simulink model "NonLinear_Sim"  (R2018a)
settings: Solver=ode113  StartTime=0.0  StopTime=40  FixedStep=Ts  MaxStep=0.005  RelTol=1e-5  EnableMultiTasking=on
InitFcn:
  | init
StopFcn:
  | pl
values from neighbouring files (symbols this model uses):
  d2r = pi/180    (= 0.0174532925199)    [init.m]    (also in LQR_Design.m)
  Ixx = 2330    [init.m]
  Iyy = 18829    [init.m]
  Izz = 18670    [init.m]
  Thr = 3.0    (= 3)    [init.m]
  x1_ini = [-1,0, -2,0, 2,0]*d2r    [init.m]
  x2_ini = [x1_ini,x2_ini]    [init.m]
  Xcg = 92.1    [init.m]
undefined symbols (not defined in the file or in its folder): Av, Bv, Cv, Dv, Kmix, Kq

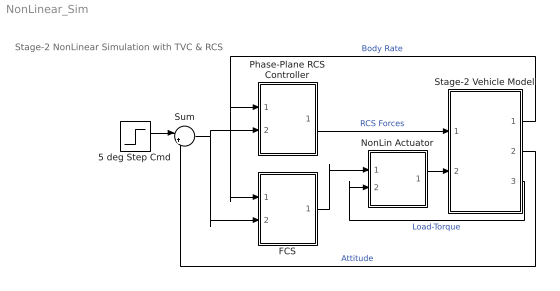
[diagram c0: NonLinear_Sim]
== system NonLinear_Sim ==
  note: Stage-2 NonLinear Simulation with TVC & RCS
  5 deg Step Cmd : Step  Time=0  Before=[0,0,0]  After=[1, 1, -1]*d2r*5  SampleTime=0
  FCS : Subsystem
  NonLin Actuator : Subsystem
  Phase-Plane RCS Controller : Subsystem
  Stage-2 Vehicle Model : Subsystem
  Sum : Sum  Inputs=|+-
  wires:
  Stage-2 Vehicle Model/1(Wb) -> FCS/1(rate), Phase-Plane RCS Controller/1(rate)  "Body Rate"
  Sum/1 -> FCS/2(atter), Phase-Plane RCS Controller/2(atter)
  Phase-Plane RCS Controller/1(f(i)) -> Stage-2 Vehicle Model/1(Frcs)  "RCS Forces"
  Stage-2 Vehicle Model/2(atti) -> Sum/2  "Attitude"
  NonLin Actuator/1(del) -> Stage-2 Vehicle Model/2(dy,dz)
  Stage-2 Vehicle Model/3(TL) -> NonLin Actuator/2(TL)  "Load-Torque"
  FCS/1(DQ,DR) -> NonLin Actuator/1(dc)
  5 deg Step Cmd/1 -> Sum/1

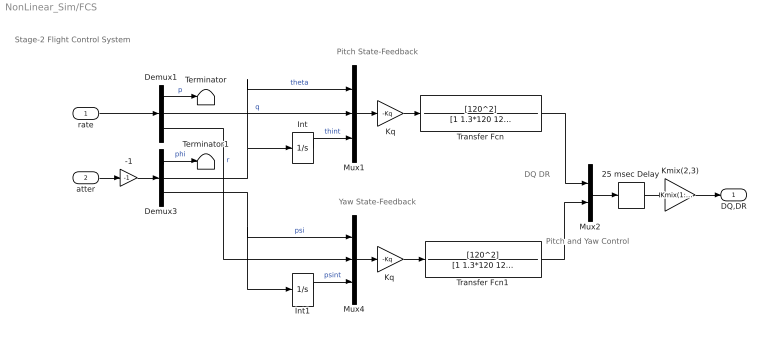
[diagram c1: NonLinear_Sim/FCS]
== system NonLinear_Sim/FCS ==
  note: Stage-2 Flight Control System
  note: DQ DR
  note: Pitch State-Feedback
  note: Yaw State-Feedback
  note: Pitch and Yaw Control
  rate : Inport
  atter : Inport  Port=2
  -1 : Gain  Gain=-1
  25 msec Delay : TransportDelay  DelayTime="[1  1]*0.025"  InitialOutput=[0 0]  PadeOrder=2
  Demux1 : Demux  Outputs=3
  Demux3 : Demux  Outputs=3
  Int : Integrator
  Int1 : Integrator
  Kmix(2,3) : Gain  Gain=Kmix(1:2,2:3)  Multiplication=Matrix(K*u)
  Kq : Gain  Gain=-Kq  Multiplication=Matrix(K*u)
  "Kq " : Gain  Gain=-Kq  Multiplication=Matrix(K*u)
  Mux1 : Mux  Inputs=3
  Mux2 : Mux  Inputs=2
  Mux4 : Mux  Inputs=3
  Terminator : Terminator
  Terminator1 : Terminator
  Transfer Fcn : TransferFcn  Numerator=[120^2]  Denominator=[1 1.3*120 120^2]
  Transfer Fcn1 : TransferFcn  Numerator=[120^2]  Denominator=[1 1.3*120 120^2]
  DQ,DR : Outport
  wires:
  25 msec Delay/1 -> Kmix(2,3)/1
  Transfer Fcn1/1 -> Mux2/2
  Kq/1 -> Transfer Fcn/1
  Mux2/1 -> 25 msec Delay/1
  "Kq "/1 -> Transfer Fcn1/1
  Transfer Fcn/1 -> Mux2/1
  Demux3/1 -> Terminator1/1  "phi"
  Demux1/1 -> Terminator/1  "p"
  Kmix(2,3)/1 -> DQ,DR/1
  rate/1 -> Demux1/1
  Demux3/2 -> Mux1/1, Int/1  "theta"
  Demux1/2 -> Mux1/2  "q"
  Int/1 -> Mux1/3  "thint"
  Int1/1 -> Mux4/3  "psint"
  Demux1/3 -> Mux4/2  "r"
  Demux3/3 -> Mux4/1, Int1/1  "psi"
  Mux1/1 -> Kq/1
  Mux4/1 -> "Kq "/1
  atter/1 -> -1/1
  -1/1 -> Demux3/1

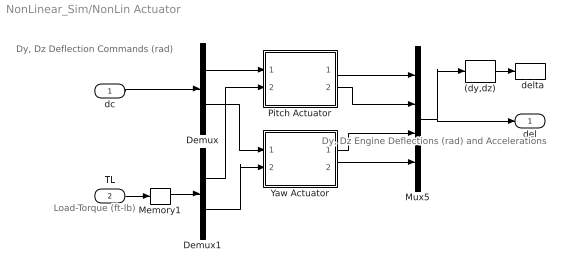
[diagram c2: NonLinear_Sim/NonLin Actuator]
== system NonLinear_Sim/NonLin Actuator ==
  note: Dy, Dz Engine Deflections (rad) and Accelerations
  note: Dy, Dz Deflection Commands (rad)
  note: Load-Torque (ft-lb)
  dc : Inport
  TL : Inport  Port=2
  "  delta" : ToWorkspace  VariableName=delta  SampleTime=-1
  (dy,dz) : Selector  InputPortWidth=4  IndexOptions=Index vector (dialog)  Indices=[1,3]  OutputSizes=1
  Demux : Demux  Outputs=2
  Demux1 : Demux  Outputs=2
  Memory1 : Memory
  Mux5 : Mux
  Pitch Actuator : Subsystem
  Yaw Actuator : Subsystem
  del : Outport
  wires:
  Pitch Actuator/1(del) -> Mux5/1
  Yaw Actuator/1(del) -> Mux5/3
  Memory1/1 -> Demux1/1
  (dy,dz)/1 -> "  delta"/1
  Demux1/1 -> Pitch Actuator/2(TL)
  Mux5/1 -> (dy,dz)/1, del/1
  Demux1/2 -> Yaw Actuator/2(TL)
  Demux/2 -> Yaw Actuator/1(delc)
  Pitch Actuator/2(ddot) -> Mux5/2
  Demux/1 -> Pitch Actuator/1(delc)
  Yaw Actuator/2(ddot) -> Mux5/4
  dc/1 -> Demux/1
  TL/1 -> Memory1/1

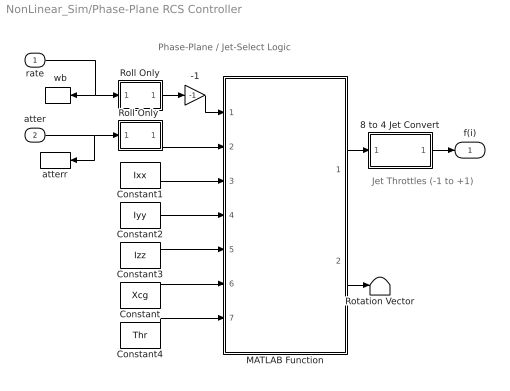
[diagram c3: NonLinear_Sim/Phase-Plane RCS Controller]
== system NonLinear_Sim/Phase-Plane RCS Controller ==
  note: Jet Throttles (-1 to +1)
  note: Phase-Plane / Jet-Select Logic
  rate : Inport
  atter : Inport  Port=2
  "  wb" : ToWorkspace  VariableName=wb  SampleTime=-1
  -1 : Gain  Gain=-1
  8 to 4 Jet Convert : Subsystem
  Constant : Constant  Value=Xcg
  Constant1 : Constant  Value=Ixx
  Constant2 : Constant  Value=Iyy
  Constant3 : Constant  Value=Izz
  Constant4 : Constant  Value=Thr
  MATLAB Function : MATLAB Function  TreatAsAtomicUnit=on
  Roll Only : Subsystem
  "Roll Only " : Subsystem
  Rotation Vector : Terminator
  atterr : ToWorkspace  VariableName=atter  SampleTime=-1
  f(i) : Outport
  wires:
  atter/1 -> atterr/1, "Roll Only "/1(w)
  "Roll Only "/1(p) -> MATLAB Function/2(Atter)
  Roll Only/1(p) -> -1/1
  -1/1 -> MATLAB Function/1(Rater)
  Constant/1 -> MATLAB Function/6(Xcg)
  rate/1 -> Roll Only/1(w), "  wb"/1
  Constant1/1 -> MATLAB Function/3(J11)
  Constant2/1 -> MATLAB Function/4(J22)
  MATLAB Function/1(fp) -> 8 to 4 Jet Convert/1(f(8))
  8 to 4 Jet Convert/1(f(4)) -> f(i)/1
  Constant3/1 -> MATLAB Function/5(J33)
  Constant4/1 -> MATLAB Function/7(Thr)
  MATLAB Function/2(eu) -> Rotation Vector/1

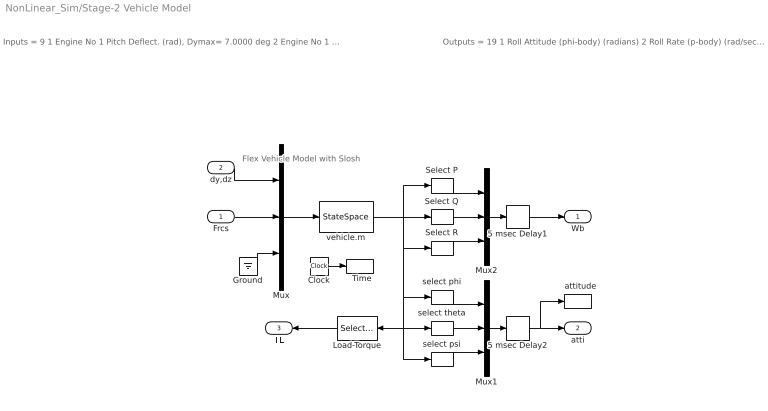
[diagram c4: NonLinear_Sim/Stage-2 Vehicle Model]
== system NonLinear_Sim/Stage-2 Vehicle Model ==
  note: Flex Vehicle Model with Slosh
  note: Outputs = 19 1 Roll Attitude (phi-body) (radians) 2 Roll Rate (p-body) (rad/sec) 3 Pitch Attitude (thet-bdy) (radians) 4 Pitch Rate (q-body) (rad/sec) 5 Yaw Attitude (psi-body) (radians) 6 Yaw Rate (r-body) (rad/sec) 7 Angle of attack, alfa, (radians) 8 Angle of sideslip, beta, (radian) 9 Change in Altitude, delta-h, (feet) 10 Forward Acceleration (V-dot) (ft/sec) 11 Cross Range Velocity (Vcr) (ft/sec) 12 Rate-Gyro # 1, Roll Rate (Body) (rad/sec) 13 Rate-Gyro # 2, Pitch Rate (Body) (rad/sec) 14 Rate-Gyro # 3, Yaw Rate (Body) (rad/sec) 15 CG Acceleration along X axis, (ft/sec^2) 16 CG Acceleration along Y axis, (ft/sec^2) 17 CG Acceleration along Z axis, (ft/sec^2) 18 Ptch Load-Torque Tly for Engine: 1,(ft-lb) 19 Yaw Load-Torque Tlz for Engine: 1,(ft-lb)
  note: Inputs = 9 1 Engine No 1 Pitch Deflect. (rad), Dymax= 7.0000 deg 2 Engine No 1 Pitch Acceleration (rad/sec^2) 3 Engine No 1 Yaw Deflect. (rad), Dzmax= 7.0000 deg 4 Engine No 1 Yaw Acceleration (rad/sec^2) 5 Throttle Input dTh/Th for Engine No 2 (-) 6 Throttle Input dTh/Th for Engine No 3 (-) 7 Throttle Input dTh/Th for Engine No 4 (-) 8 Throttle Input dTh/Th for Engine No 5 (-) 9 Wind Gust Azim, Elev Angles=( 45.0 90.0) (deg)
  Frcs : Inport
  dy,dz : Inport  Port=2
  "  Time" : ToWorkspace  VariableName=tim  SampleTime=-1
  "  attitude" : ToWorkspace  VariableName=atti  SampleTime=-1
  5 msec Delay1 : TransportDelay  DelayTime=0.005*[1 1 1]  InitialOutput=[0 0 0]  PadeOrder=2
  5 msec Delay2 : TransportDelay  DelayTime=0.005*[1 1 1]  InitialOutput=x1_ini([1,3,5])  PadeOrder=2
  Clock : Clock
  Ground : Ground
  Load-Torque : Selector  InputPortWidth=19  IndexOptions=Index vector (dialog)  Indices=[18, 19]  OutputSizes=1
  Mux : Mux  Inputs=[4,4,1]
  Mux1 : Mux  Inputs=3
  Mux2 : Mux  Inputs=3
  Select P : Selector  InputPortWidth=19  IndexOptions=Index vector (dialog)  Indices=[12]  OutputSizes=1
  Select Q : Selector  InputPortWidth=19  IndexOptions=Index vector (dialog)  Indices=[13]  OutputSizes=1
  Select R : Selector  InputPortWidth=19  IndexOptions=Index vector (dialog)  Indices=[14]  OutputSizes=1
  select phi : Selector  InputPortWidth=19  IndexOptions=Index vector (dialog)  Indices=[1]  OutputSizes=1
  select psi : Selector  InputPortWidth=19  IndexOptions=Index vector (dialog)  Indices=[5]  OutputSizes=1
  select theta : Selector  InputPortWidth=19  IndexOptions=Index vector (dialog)  Indices=[3]  OutputSizes=1
  vehicle.m : StateSpace  A=Av  B=Bv  C=Cv  D=Dv  InitialCondition=x2_ini
  Wb : Outport
  atti : Outport  Port=2
  TL : Outport  Port=3
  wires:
  5 msec Delay2/1 -> "  attitude"/1, atti/1
  Mux2/1 -> 5 msec Delay1/1
  Mux/1 -> vehicle.m/1
  dy,dz/1 -> Mux/1
  Ground/1 -> Mux/3
  Frcs/1 -> Mux/2
  Clock/1 -> "  Time"/1
  Load-Torque/1 -> TL/1
  select psi/1 -> Mux1/3
  select phi/1 -> Mux1/1
  vehicle.m/1 -> select psi/1, Load-Torque/1, select theta/1, select phi/1, Select R/1, Select P/1, Select Q/1
  Select Q/1 -> Mux2/2
  select theta/1 -> Mux1/2
  Select R/1 -> Mux2/3
  Select P/1 -> Mux2/1
  Mux1/1 -> 5 msec Delay2/1
  5 msec Delay1/1 -> Wb/1

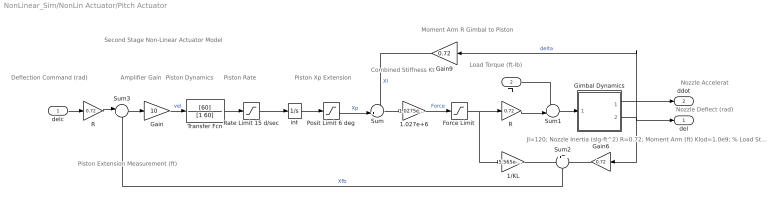
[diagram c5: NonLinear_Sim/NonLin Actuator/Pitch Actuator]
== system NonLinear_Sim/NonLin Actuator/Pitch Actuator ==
  note: Piston Extension Measurement (ft)
  note: Moment Arm R Gimbal to Piston
  note: Second Stage Non-Linear Actuator Model
  note: Piston Rate
  note: Amplifier Gain
  note: Nozzle Deflect (rad)
  note: Nozzle Accelerat
  note: Piston Dynamics
  note: Combined Stiffness Kt
  note: Piston Xp Extension
  note: Deflection Command (rad)
  note: Load Torque (ft-lb)
  note: Jl=120; Nozzle Inertia (slg-ft^2) R=0.72; Moment Arm (ft) Klod=1.0e9; % Load Stiffness Kact=2.4e6; % Piston Stiffness Kbck=1.13e6; % Backup Structure Stiffn Kti=(1/Klod)+(1/Kact)+(1/Kbck); Kt=1/Kti; % Combined Structural Stiffness Ka=8; % Amplifier Gain
  delc : Inport
  TL : Inport  Port=2
  1.027e+6 : Gain  Gain=1.0275e+6
  1/KL : Gain  Gain=5.565e-07
  Force Limit : Saturate  UpperLimit=4000  LowerLimit=-4000
  Gain : Gain  Gain=10
  Gain6 : Gain  Gain=0.72
  Gain9 : Gain  Gain=0.72
  Gimbal Dynamics : Subsystem
  Posit Limit 6 deg : Saturate  UpperLimit=0.075  LowerLimit=-0.075
  R : Gain  Gain=0.72
  "R " : Gain  Gain=0.72
  Rate Limit 15 d/sec : Saturate  UpperLimit=0.125  LowerLimit=-0.125
  Sum : Sum  Inputs=-+|
  Sum1 : Sum  Inputs=++|
  Sum2 : Sum  Inputs=+|+
  Sum3 : Sum  Inputs=|+-
  Transfer Fcn : TransferFcn  Numerator=[60]  Denominator=[1 60]
  int : Integrator
  del : Outport
  ddot : Outport  Port=2
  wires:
  Sum2/1 -> Sum3/2  "Xfb"
  Gimbal Dynamics/2(" delta") -> Gain6/1, del/1, Gain9/1  "delta"
  "R "/1 -> Sum1/2
  Force Limit/1 -> 1/KL/1, "R "/1
  delc/1 -> R/1
  R/1 -> Sum3/1
  TL/1 -> Sum1/1
  int/1 -> Posit Limit 6 deg/1
  Sum/1 -> 1.027e+6/1
  Sum3/1 -> Gain/1
  Gain/1 -> Transfer Fcn/1  "vel"
  Rate Limit 15 d/sec/1 -> int/1
  Gain6/1 -> Sum2/2
  1.027e+6/1 -> Force Limit/1  "Force"
  Gain9/1 -> Sum/1  "Xl"
  1/KL/1 -> Sum2/1
  Posit Limit 6 deg/1 -> Sum/2  "Xp"
  Gimbal Dynamics/1(Axel) -> ddot/1
  Sum1/1 -> Gimbal Dynamics/1(Tin)
  Transfer Fcn/1 -> Rate Limit 15 d/sec/1

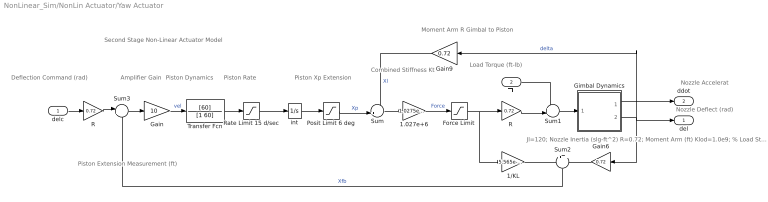
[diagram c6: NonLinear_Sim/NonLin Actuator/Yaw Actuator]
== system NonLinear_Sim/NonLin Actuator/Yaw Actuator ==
  note: Piston Extension Measurement (ft)
  note: Moment Arm R Gimbal to Piston
  note: Second Stage Non-Linear Actuator Model
  note: Piston Rate
  note: Amplifier Gain
  note: Nozzle Deflect (rad)
  note: Nozzle Accelerat
  note: Piston Dynamics
  note: Combined Stiffness Kt
  note: Piston Xp Extension
  note: Deflection Command (rad)
  note: Load Torque (ft-lb)
  note: Jl=120; Nozzle Inertia (slg-ft^2) R=0.72; Moment Arm (ft) Klod=1.0e9; % Load Stiffness Kact=2.4e6; % Piston Stiffness Kbck=1.13e6; % Backup Structure Stiffn Kti=(1/Klod)+(1/Kact)+(1/Kbck); Kt=1/Kti; % Combined Structural Stiffness Ka=8; % Amplifier Gain
  delc : Inport
  TL : Inport  Port=2
  1.027e+6 : Gain  Gain=1.0275e+6
  1/KL : Gain  Gain=5.565e-07
  Force Limit : Saturate  UpperLimit=4000  LowerLimit=-4000
  Gain : Gain  Gain=10
  Gain6 : Gain  Gain=0.72
  Gain9 : Gain  Gain=0.72
  Gimbal Dynamics : Subsystem
  Posit Limit 6 deg : Saturate  UpperLimit=0.075  LowerLimit=-0.075
  R : Gain  Gain=0.72
  "R " : Gain  Gain=0.72
  Rate Limit 15 d/sec : Saturate  UpperLimit=0.125  LowerLimit=-0.125
  Sum : Sum  Inputs=-+|
  Sum1 : Sum  Inputs=++|
  Sum2 : Sum  Inputs=+|+
  Sum3 : Sum  Inputs=|+-
  Transfer Fcn : TransferFcn  Numerator=[60]  Denominator=[1 60]
  int : Integrator
  del : Outport
  ddot : Outport  Port=2
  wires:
  Sum2/1 -> Sum3/2  "Xfb"
  Gimbal Dynamics/2(" delta") -> Gain6/1, del/1, Gain9/1  "delta"
  "R "/1 -> Sum1/2
  Force Limit/1 -> 1/KL/1, "R "/1
  delc/1 -> R/1
  R/1 -> Sum3/1
  TL/1 -> Sum1/1
  int/1 -> Posit Limit 6 deg/1
  Sum/1 -> 1.027e+6/1
  Sum3/1 -> Gain/1
  Gain/1 -> Transfer Fcn/1  "vel"
  Rate Limit 15 d/sec/1 -> int/1
  Gain6/1 -> Sum2/2
  1.027e+6/1 -> Force Limit/1  "Force"
  Gain9/1 -> Sum/1  "Xl"
  1/KL/1 -> Sum2/1
  Posit Limit 6 deg/1 -> Sum/2  "Xp"
  Gimbal Dynamics/1(Axel) -> ddot/1
  Sum1/1 -> Gimbal Dynamics/1(Tin)
  Transfer Fcn/1 -> Rate Limit 15 d/sec/1

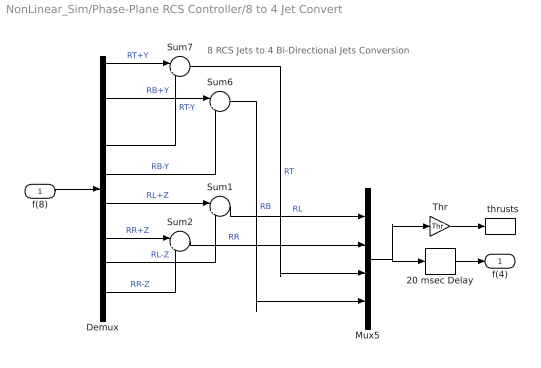
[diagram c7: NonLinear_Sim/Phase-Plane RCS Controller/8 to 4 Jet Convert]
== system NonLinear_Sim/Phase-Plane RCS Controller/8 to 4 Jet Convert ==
  note: 8 RCS Jets to 4 Bi-Directional Jets Conversion
  f(8) : Inport
  "  thrusts" : ToWorkspace  VariableName=Jets  SampleTime=-1
  20 msec Delay : TransportDelay  DelayTime="[1  1  1  1]*0.020"  InitialOutput="[0  0  0  0]"  PadeOrder=2
  Demux : Demux  Outputs=8
  Mux5 : Mux
  Sum{1..2,6..7} (4 alike) : Sum  Inputs=|+-
  Thr : Gain  Gain=Thr
  f(4) : Outport
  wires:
  f(8)/1 -> Demux/1
  Mux5/1 -> 20 msec Delay/1, Thr/1
  Demux/7 -> Sum1/2  "RL-Z"
  Demux/6 -> Sum2/1  "RR+Z"
  Demux/1 -> Sum7/1  "RT+Y"
  Sum6/1 -> Mux5/4  "RB"
  Demux/5 -> Sum1/1  "RL+Z"
  Demux/8 -> Sum2/2  "RR-Z"
  Sum7/1 -> Mux5/3  "RT"
  Demux/3 -> Sum7/2  "RT-Y"
  Demux/2 -> Sum6/1  "RB+Y"
  Demux/4 -> Sum6/2  "RB-Y"
  Sum1/1 -> Mux5/1  "RL"
  Sum2/1 -> Mux5/2  "RR"
  20 msec Delay/1 -> f(4)/1
  Thr/1 -> "  thrusts"/1

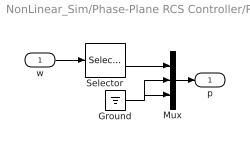
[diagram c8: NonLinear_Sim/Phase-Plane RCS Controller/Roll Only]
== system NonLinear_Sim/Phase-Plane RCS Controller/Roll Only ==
  w : Inport
  Ground : Ground
  Mux : Mux  Inputs=3
  Selector : Selector  InputPortWidth=3  IndexOptions=Index vector (dialog)  Indices=[1]  OutputSizes=1
  p : Outport
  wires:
  w/1 -> Selector/1
  Mux/1 -> p/1
  Selector/1 -> Mux/1
  Ground/1 -> Mux/3, Mux/2

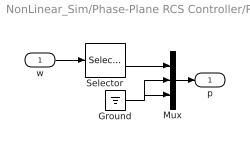
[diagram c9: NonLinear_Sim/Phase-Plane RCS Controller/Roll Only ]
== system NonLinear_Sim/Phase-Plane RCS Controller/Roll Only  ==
  w : Inport
  Ground : Ground
  Mux : Mux  Inputs=3
  Selector : Selector  InputPortWidth=3  IndexOptions=Index vector (dialog)  Indices=[1]  OutputSizes=1
  p : Outport
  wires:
  w/1 -> Selector/1
  Mux/1 -> p/1
  Selector/1 -> Mux/1
  Ground/1 -> Mux/3, Mux/2

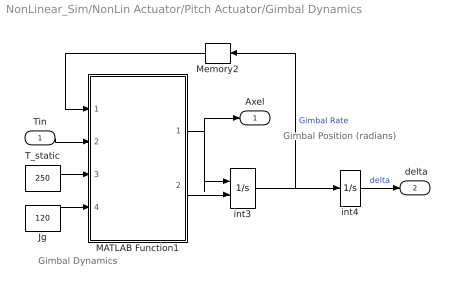
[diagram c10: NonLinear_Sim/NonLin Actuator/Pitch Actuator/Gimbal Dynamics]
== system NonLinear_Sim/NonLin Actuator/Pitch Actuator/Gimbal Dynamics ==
  note: Gimbal Position (radians)
  note: Gimbal Dynamics
  Tin : Inport
  Jg : Constant  Value=120
  MATLAB Function1 : MATLAB Function  TreatAsAtomicUnit=on
  Memory2 : Memory
  T_static : Constant  Value=250
  int3 : Integrator  ExternalReset=rising
  int4 : Integrator
  Axel : Outport
  " delta" : Outport  Port=2
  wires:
  MATLAB Function1/2(Rvel) -> int3/2
  int4/1 -> " delta"/1  "delta"
  int3/1 -> int4/1, Memory2/1  "Gimbal Rate"
  Tin/1 -> MATLAB Function1/2(Tin)
  T_static/1 -> MATLAB Function1/3(Tst)
  MATLAB Function1/1(Axel) -> Axel/1, int3/1
  Jg/1 -> MATLAB Function1/4(Jg)
  Memory2/1 -> MATLAB Function1/1(Rate)

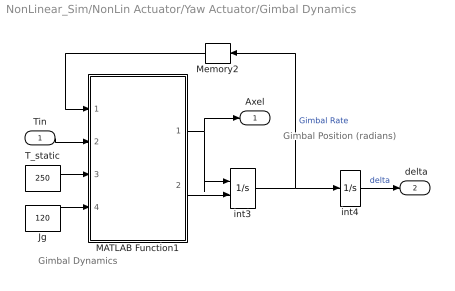
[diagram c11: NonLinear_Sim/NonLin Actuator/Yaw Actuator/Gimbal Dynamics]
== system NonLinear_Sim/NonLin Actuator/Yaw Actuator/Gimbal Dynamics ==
  note: Gimbal Position (radians)
  note: Gimbal Dynamics
  Tin : Inport
  Jg : Constant  Value=120
  MATLAB Function1 : MATLAB Function  TreatAsAtomicUnit=on
  Memory2 : Memory
  T_static : Constant  Value=250
  int3 : Integrator  ExternalReset=rising
  int4 : Integrator
  Axel : Outport
  " delta" : Outport  Port=2
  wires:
  MATLAB Function1/2(Rvel) -> int3/2
  int4/1 -> " delta"/1  "delta"
  int3/1 -> int4/1, Memory2/1  "Gimbal Rate"
  Tin/1 -> MATLAB Function1/2(Tin)
  T_static/1 -> MATLAB Function1/3(Tst)
  MATLAB Function1/1(Axel) -> Axel/1, int3/1
  Jg/1 -> MATLAB Function1/4(Jg)
  Memory2/1 -> MATLAB Function1/1(Rate)

== matlab function NonLinear_Sim/NonLin Actuator/Yaw Actuator/Gimbal 
Dynamics/MATLAB Function1 ==
function [Axel,Rvel] = Gimbal(Rate,Tin,Tst,Jg)    
% Gimbal Friction Dynamics
% Tin:  Input Torque (ft-lb)
% Rate: Gimbal Rate (rad/sec)
% Tfr:  Gimbal Friction Torque (ft-lb)
% axel: Gimbal Acceleration (ft/sec2)
% Tst:  Gimbal Static Friction Torq (ft-lb)
% Jg:   Gimbal Inertia (slg-ft^2)

if abs(Rate)<0.01                     % If Not Moving Much
    if abs(Tin)>Tst*1.05              % Exceeds Stiction, Start Moving
        Tfr=Tst*sign(Tin);            % Friction Torque resist motion
        Axel=(Tin-Tfr)/Jg;            % Gimbal Acceleration
        Rvel=0;
    else                              % Stop the Motion
        Axel=0;
        Tfr=0;                        % No Frict when not moving
        Rvel=1;                       % Reset Velocity to Zero
    end
    
else                                  % Gimbal is Fast Enough
    Tfr=Tst*sign(Rate);               % Friction Torque resist motion
    Axel=(Tin-Tfr)/Jg;                % Gimbal Acceleration
    Rvel=0;
end

== matlab function NonLinear_Sim/Phase-Plane
RCS Controller/MATLAB Function ==
function [fp, eu]= Phase_Plane(Rater,Atter, J11,J22,J33, Xcg,Thr)    
% Phase-Plane Logic for RCS jets
% Rater: Rate Error in (deg/sec)
% Atter: Attitude Error in (deg)

% Define Phase-Plane Logic Parameters in (deg)
r2d=180/pi;
nt=8;                                                    % Number of Jets
cg2= [Xcg, 0.0, 0.0]';                                   % CG Location
ang_acl     = Thr*160*[6/J11, 20/J22, 20/J33];
att_deadband= [1, 1, 1]*0.5; 
kledge      = [1, 1, 1]*1.2; 
rate_lim    = [1, 1, 1]*7.0; 
low_rate_lim= rate_lim*0.31;

% RCS Thruster Directions ----------------------------------------------
Jdir= zeros(3,nt); Jloc=Jdir;
Jdir(:, 1)= [0.0,  +1.0,   0.0]';                         % Top   +Y
Jdir(:, 2)= [0.0,  +1.0,   0.0]';                         % Botm  +Y
Jdir(:, 3)= [0.0,  -1.0,   0.0]';                         % Top   -Y
Jdir(:, 4)= [0.0,  -1.0,   0.0]';                         % Botm  -Y
Jdir(:, 5)= [0.0,   0.0,  +1.0]';                         % Left  +Z
Jdir(:, 6)= [0.0,   0.0,  +1.0]';                         % Right +Z
Jdir(:, 7)= [0.0,   0.0,  -1.0]';                         % Left  -Z
Jdir(:, 8)= [0.0,   0.0,  -1.0]';                         % Right -Z

% RCS Thruster Locations -----------------------------------------------
Jloc(:, 1) = [83,  0.0, -3.5]';                           % Top   +Y
Jloc(:, 2) = [83,  0.0, +3.5]';                           % Botm  +Y
Jloc(:, 3) = [83,  0.0, -3.5]';                           % Top   -Y
Jloc(:, 4) = [83,  0.0, +3.5]';                           % Botm  -Y
Jloc(:, 5) = [83, -3.5,  0.0]';                           % Left  +Z
Jloc(:, 6) = [83, +3.5,  0.0]';                           % Right +Z
Jloc(:, 7) = [83, -3.5,  0.0]';                           % Left  -Z
Jloc(:, 8) = [83, +3.5,  0.0]';                           % Right -Z

rat_err= Rater*r2d;                                    % Convert to (deg)
att_err= Atter*r2d;
Cnt= [0;0;0];                                          % Control to JetSel

for iax=1:3
    sign_rat_err= sign(rat_err(iax)+1.0e-8);
    x1 = sign_rat_err*att_err(iax);
    x2 = abs(rat_err(iax));
    ang_acl_gain= 2*ang_acl(iax);
    curve = rat_err(iax)^2/ang_acl_gain;
    
    sw1= -curve + att_deadband(iax);
    sw2= -(curve + (kledge(iax)*att_deadband(iax)));
    sw3= rate_lim(iax);
    sw5= low_rate_lim(iax);
    
    if ((x1>sw1) || (x2>sw3)), Cnt(iax)= -sign_rat_err; % Region 1
    elseif (x1 >= sw2), Cnt(iax)= 0;                    % Region 2
    elseif (x2 < sw5), Cnt(iax)= sign_rat_err;          % Region 3
    else, Cnt(iax)= 0;  
    end
end

% Select Jets
if abs(Cnt)>0, eu= Cnt/sqrt(Cnt'*Cnt);                  % Direction Unit vect
else, eu=Cnt; end
fp= Jet_Select_dot(-eu,4, nt,Thr,cg2,Jloc,Jdir);        % Get Thruster Forces

function fp= Jet_Select_dot(eu,Imax, nt,Thr,cg2,Jloc,Jdir)
% fp= Jet_Select_dot(eu,nt,Thr,Jloc,Jdir,Imax)
% Compute the thrust force vector (fp)
% Inputs
% eu(3) : ACS error unit vector
% nt    : number of jets
% Thr   : Thrust in (lb)
% Jloc  : Jet Locations 
% Jdir  : Thrust directions
% Imax  : Max number of Thrusters to select
% J     : Vehicle MOI matrix (3x3)
% cg(3) : CG location
% Outputs
% fp(nt): Thrusts vector (nt)

if sqrt(eu'*eu)<0.9, fp=zeros(nt,1); return; end    % Direct must be unit vect

tm= Thr*ones(1,nt);
vt= zeros(3,nt); pf= zeros(nt,1); sf=pf;

% Select the most dominant jets from all of them
for i=1:nt
    ln= (Jloc(:,i) - cg2);                          % Moment arms
    vt(:,i)= tm(i)*cross(ln,Jdir(:,i));             % Moments Matrix using all jets
    pf(i) = dot(vt(:,i),eu);                        % Moment dotted with maneuv direct
end

f2=pf;
for i=1:(nt/2)
    [mf,sf(i)]=max(f2); f2(sf(i))=0;                % Identify the strongest half
end
pf= pf/pf(sf(1));                                   % Normlz relative to strongest

% Select Imax jets among the strongest
Isel=1;                                             % First, select the strongest
for i=1:Imax-1
    if pf(sf(i+1))>0.72; Isel=Isel+1; end            % 70% contrib, choose one more jet to Imax
end

fp= zeros(nt,1);                                    % Initially zero all jets
for i=1:nt
    for j=1:Isel
        if i==sf(j); fp(i)=1; end                   % Turn on the selected jet force
    end
end

== matlab function NonLinear_Sim/NonLin Actuator/Pitch Actuator/Gimbal 
Dynamics/MATLAB Function1 ==
function [Axel,Rvel] = Gimbal(Rate,Tin,Tst,Jg)    
% Gimbal Friction Dynamics
% Tin:  Input Torque (ft-lb)
% Rate: Gimbal Rate (rad/sec)
% Tfr:  Gimbal Friction Torque (ft-lb)
% axel: Gimbal Acceleration (ft/sec2)
% Tst:  Gimbal Static Friction Torq (ft-lb)
% Jg:   Gimbal Inertia (slg-ft^2)

if abs(Rate)<0.01                     % If Not Moving Much
    if abs(Tin)>Tst*1.05              % Exceeds Stiction, Start Moving
        Tfr=Tst*sign(Tin);            % Friction Torque resist motion
        Axel=(Tin-Tfr)/Jg;            % Gimbal Acceleration
        Rvel=0;
    else                              % Stop the Motion
        Axel=0;
        Tfr=0;                        % No Frict when not moving
        Rvel=1;                       % Reset Velocity to Zero
    end
    
else                                  % Gimbal is Fast Enough
    Tfr=Tst*sign(Rate);               % Friction Torque resist motion
    Axel=(Tin-Tfr)/Jg;                % Gimbal Acceleration
    Rvel=0;
end
